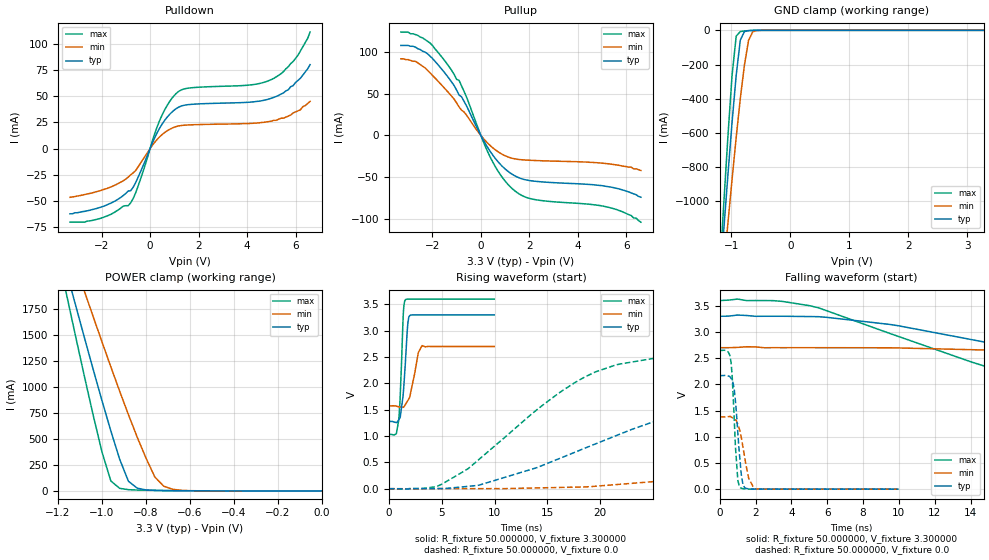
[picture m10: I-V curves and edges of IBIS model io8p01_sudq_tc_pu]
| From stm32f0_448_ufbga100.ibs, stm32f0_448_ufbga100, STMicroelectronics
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|   Model io8p01_sudq_tc_pu
[Model]  io8p01_sudq_tc_pu
Model_type I/O
Polarity   Non-Inverting
Enable   Active-Low
Vinl =   0.990000V
Vinh =   2.310000V
Vmeas =  1.650000V
Cref =   50.000000pF
Rref =   100.000000M
Vref =   0.0V
C_comp   1.329900pF   1.255600pF   1.431200pF
[Temperature Range]   25.000000   0.125000k   -40.000000
[Pullup Reference]   3.300000V   2.700000V   3.600000V
[Pulldown Reference]   0.0V   0.0V   0.0V
[POWER Clamp Reference]   3.300000V   2.700000V   3.600000V
[GND Clamp Reference]   0.0V   0.0V   0.0V
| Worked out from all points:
|   slope of the pulldown table from 0 to 0.495 V, typ, clamps not added: 21.3 ohm
|   slope of the pullup table from 0 to 0.495 V, typ, clamps not added: 20.9 ohm
|   GND clamp passes 1 mA (typ) near -0.67 V on its own axis
|   POWER clamp passes 1 mA (typ) near -0.60 V on its own axis
|   rising waveform, R_fixture 50.000000, V_fixture 3.300000: 20-80 % time 415ps typ, 658ps min, 304ps max; typ from 1.28 V to 3.3 V
|   rising waveform, R_fixture 50.000000, V_fixture 0.0: 20-80 % time 18.4ns typ, 45.6ns min, 10.1ns max; typ from 0.001 V to 2.17 V
|   falling waveform, R_fixture 50.000000, V_fixture 3.300000: 20-80 % time 25.8ns typ, 44.2ns min, 16.3ns max; typ from 3.3 V to 1.28 V
|   falling waveform, R_fixture 50.000000, V_fixture 0.0: 20-80 % time 301ps typ, 443ps min, 235ps max; typ from 2.17 V to 0.001 V
[Pulldown]
|Voltage   I(typ)   I(min)   I(max)
-3.3V     -62mA      -46.3mA    -70mA
-2.1V     -56.2mA    -40.3mA    -66.8mA
-800mV    -40.05mA   -24.9mA    -51.58mA
-500mV    -27.57mA   -17.6mA    -36.07mA
400mV     19.71mA    11.36mA    27.01mA
700mV     29.83mA    16.93mA    40.97mA
1.1V      38.46mA    21.2mA     53.02mA
1.6V      41.98mA    22.62mA    57.7mA
4.1V      44.26mA    24mA       60.59mA
5V        48mA       26.2mA     65.8mA
5.9V      60mA       34mA       83mA
6.6V      80mA       45mA       111mA
[Pullup]
|Voltage   I(typ)   I(min)   I(max)
-3.3V     108mA      92mA       124mA
-2.7V     106mA      89mA       121mA
-2.2V     98mA       78.1mA     113mA
-1.4V     71.8mA     53.5mA     86.1mA
-900mV    48.5mA     34.23mA    66.14mA
-700mV    41.33mA    28.36mA    53.31mA
400mV     -19.77mA   -12.52mA   -26.8mA
900mV     -37.48mA   -22.89mA   -50.99mA
1.4V      -48.39mA   -28.06mA   -66.43mA
2.2V      -54.79mA   -29.98mA   -76.75mA
5.3V      -61.6mA    -34.1mA    -86.4mA
6.6V      -74mA      -42mA      -104mA
[GND_clamp]
|Voltage   I(typ)   I(min)   I(max)
-3.3V     -9.739A    -9.975A    -9.587A
-1.2V     -1.489A    -1.65A     -1.416A
-1.13V    -1.162A    -1.385A    -1.009A
-1.06V    -842.2mA   -1.125A    -616.9mA
-990mV    -537.1mA   -870.1mA   -263mA
-920mV    -262.4mA   -625.3mA   -33.96mA
-850mV    -56.94mA   -397.4mA   -7.08mA
-780mV    -7.011mA   -202.2mA   -3.71mA
-710mV    -1.778mA   -58.23mA   -1.736mA
-640mV    -550uA     -8.783mA   -542.4uA
-570mV    -109.8uA   -1.292mA   -86.89uA
3.28V     0A         0A         0A
[POWER_clamp]
|Voltage   I(typ)   I(min)   I(max)
-3.28V    9.897A     9.838A     9.594A
-1.16V    2.103A     2.419A     1.88A
-1.12V    1.788A     2.17A      1.488A
-1.08V    1.476A     1.923A     1.102A
-1V       868.2mA    1.435A     373.1mA
-960mV    578.3mA    1.196A     96.08mA
-880mV    93.25mA    734.2mA    12.03mA
-840mV    26.31mA    517.4mA    8.576mA
-760mV    5.12mA     134mA      5.134mA
-720mV    3.368mA    46.35mA    3.823mA
-600mV    1.018mA    2.575mA    1.086mA
0V        0A         0A         0A
[Ramp]
| variable   typ   min   max
dV/dt_r  1.30013/18.38759n   0.82685/45.50659n   1.58870/10.13811n
dV/dt_f  1.21404/25.72381n   0.67656/44.12572n   1.54164/16.31478n
R_load = 50.000000
[Rising Waveform]
R_fixture= 50.000000
V_fixture= 3.300000
V_fixture_min= 2.700000
V_fixture_max= 3.600000
|time   V(typ)   V(min)   V(max)
0s        1.277V     1.572V     1.031V
700.7ps   1.258V     1.568V     1.044V
940.9ps   1.31V      1.555V     1.309V
1.061ns   1.349V     1.55V      1.702V
1.381ns   1.858V     1.546V     3.369V
1.582ns   2.46V      1.605V     3.589V
1.902ns   3.263V     1.709V     3.6V
2.783ns   3.3V       2.579V     3.6V
3.143ns   3.3V       2.717V     3.6V
9.97ns    3.3V       2.7V       3.6V
[Rising Waveform]
R_fixture= 50.000000
V_fixture= 0.0
V_fixture_min= 0.0
V_fixture_max= 0.0
|time   V(typ)   V(min)   V(max)
0s        1.014mV    1.116mV    973.4uV
5.005ns   4.509mV    2.878mV    86.36mV
8.509ns   67.44mV    3.12mV     554mV
15.52ns   523.4mV    22.26mV    1.731V
19.52ns   849.3mV    47.73mV    2.216V
25.53ns   1.305V     143.4mV    2.489V
33.53ns   1.765V     271mV      2.592V
47.55ns   2.063V     578mV      2.637V
88.59ns   2.166V     1.194V     2.649V
249.2ns   2.168V     1.379V     2.649V
[Falling Waveform]
R_fixture= 50.000000
V_fixture= 3.300000
V_fixture_min= 2.700000
V_fixture_max= 3.600000
|time   V(typ)   V(min)   V(max)
0s        3.3V       2.7V       3.6V
3.003ns   3.3V       2.7V       3.598V
5.506ns   3.292V     2.7V       3.462V
14.51ns   2.825V     2.658V     2.377V
21.02ns   2.42V      2.556V     1.792V
29.03ns   2.031V     2.4V       1.343V
38.54ns   1.7V       2.218V     1.13V
55.06ns   1.41V      1.956V     1.055V
105.6ns   1.281V     1.626V     1.03V
249.2ns   1.277V     1.572V     1.031V
[Falling Waveform]
R_fixture= 50.000000
V_fixture= 0.0
V_fixture_min= 0.0
V_fixture_max= 0.0
|time   V(typ)   V(min)   V(max)
0s        2.168V     1.379V     2.649V
620.6ps   2.122V     1.383V     2.45V
700.7ps   2.076V     1.364V     2.13V
820.8ps   1.879V     1.335V     1.257V
1.001ns   1.131V     1.243V     224.3mV
1.161ns   446.2mV    1.059V     27.44mV
1.381ns   33.87mV    633.5mV    6.297mV
1.622ns   6.705mV    205.1mV    3.679mV
1.942ns   1.889mV    4.742mV    3.498mV
9.97ns    1.014mV    1.116mV    973.4uV
